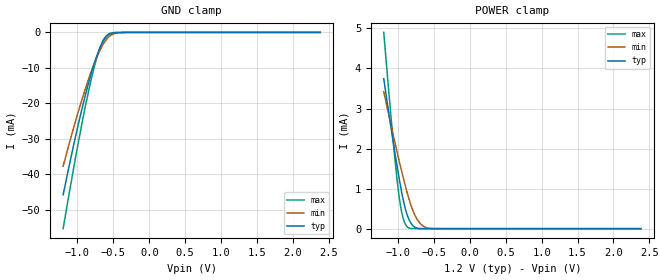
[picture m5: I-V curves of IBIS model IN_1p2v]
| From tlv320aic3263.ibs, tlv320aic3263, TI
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|   IN_1p2v
[Model]   IN_1p2v
Model_type   Input
Vinl = 1.08
Vinh = 0.12
|   typ   min   max
C_comp   1.095pF   1.082pF   1.133pF
[Voltage Range]   1.2   1.1   1.3
[Temperature Range]   27   125   -40
[Power Clamp Reference]   1.2   1.1   1.3
[GND Clamp Reference]   -0   -0   -0
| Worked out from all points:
|   GND clamp passes 1 mA (typ) near -0.58 V on its own axis
|   POWER clamp passes 1 mA (typ) near -0.96 V on its own axis
[GND Clamp]
|   Voltage   I(typ)   I(min)   I(max)
-1.2V     -45.78mA   -37.73mA   -55.33mA
-1.11V    -37.06mA   -30.96mA   -44.72mA
-984mV    -25.55mA   -22.02mA   -30.58mA
-894mV    -18.01mA   -16.12mA   -21.24mA
-822mV    -12.53mA   -11.79mA   -14.42mA
-750mV    -7.751mA   -7.917mA   -8.472mA
-696mV    -4.78mA    -5.405mA   -4.842mA
-642mV    -2.508mA   -3.332mA   -2.212mA
-588mV    -1.053mA   -1.79mA    -741uA
-480mV    -90.52uA   -311.7uA   -33.57uA
-300mV    -348.8nA   -5.721uA   -17.65nA
2.382V    0A         0A         0A
[POWER Clamp]
|   Voltage   I(typ)   I(min)   I(max)
-1.2V     3.742mA    3.419mA    4.901mA
-1.074V   2.231mA    2.387mA    2.298mA
-1.002V   1.428mA    1.82mA     1.03mA
-966mV    1.06mA     1.547mA    562.3uA
-930mV    731.2uA    1.283mA    261.4uA
-894mV    461.8uA    1.032mA    95.61uA
-858mV    267uA      798.5uA    24.84uA
-804mV    94.08uA    498uA      2.263uA
-732mV    11.82uA    224.2uA    76.87nA
-660mV    950.1nA    77.55uA    837.8pA
-570mV    32.74nA    10.88uA    0A
2.382V    0A         0A         0A
